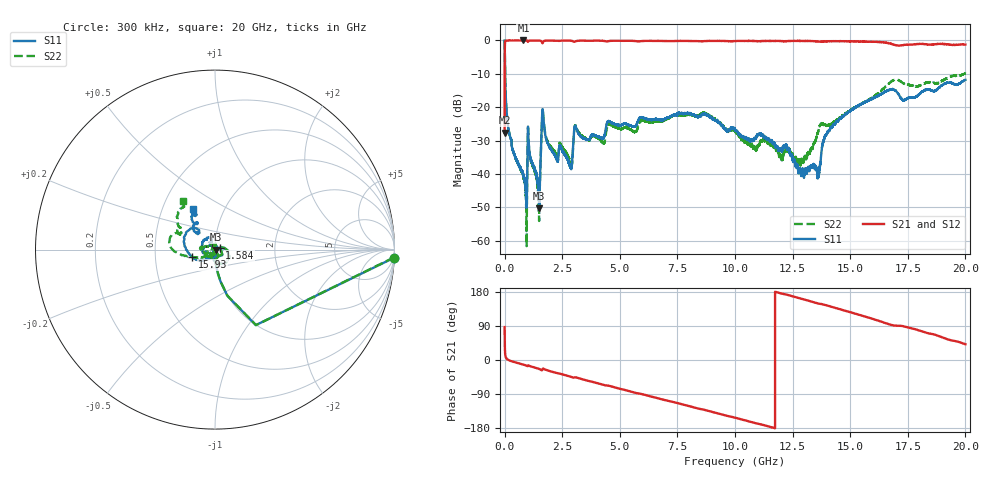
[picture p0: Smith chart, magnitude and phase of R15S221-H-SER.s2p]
!{R15S221}
!Johanson Technology Inc.
!www.johansontechnology.com
!Test Board Conditions:
!Substrate Type  RO4350B
!Substrate Thickness  20 mil
!Substrate Dk  3.66
!TL Type: GCPW
!TL Trace Width  34 mil
!TL Gap  10 mil
!Electrode orientation  Horizontal
!DUT TOPOLOGY	SERIES
!Mounting Pad LxW  26x52 mil
! Created Sat Feb  6 14:22:14 2021
# hz S ma R 50
! 2 Port Network Data from SP1.SP block
! freq  magS11  angS11  magS21  angS21  magS12  angS12  magS22  angS22
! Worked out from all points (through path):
!   20001 points, 300 kHz to 20 GHz, reference 50 ohm
!   highest |S21| = 0.00 dB at 816.3 MHz (marker M1); lowest = -27.7 dB at 300 kHz (marker M2)
!   group delay of S21, straight-line fit = 44.1 ps
!   lowest |S11| = -50.2 dB at 1.501 GHz (marker M3), VSWR 1.01, Z = 50.3 - j0.117 ohm
!   |S11| at or under -10 dB: 21.74 MHz to end of sweep
!   |S22| runs from -61.6 to 0.0 dB; largest |S21 - S12| = 0.014
!   S11 on the Smith chart (normalised r, x): 300 kHz: 2, -44; 1.584 GHz: 1.05, +0.02; 15.93 GHz: 0.77, -0.07; 20 GHz: 0.71, +0.34
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300000  0.9983 -2.6  0.0414 86.9  0.0415 87.4  0.9969 -2.5
1.073e8  0.06955 -87.6  0.9969 2.2  0.9969 2.2  0.06989 -87.4
4.003e8  0.02077 -94.3  0.9994 -5.1  0.999 -5.1  0.0206 -95.1
8.163e8  0.00948 -97.8  0.9999 -12.3  0.9984 -12.2  0.00937 -106.7
8.923e8  0.007055 -97.5  0.9982 -13.6  0.9984 -13.6  0.006714 -109.6
1.0893e9  0.02004 -101.3  0.9963 -16.1  0.9959 -16.0  0.01927 -103.2
1.5013e9  0.003086 -22.2  0.9954 -23.6  0.9954 -23.7  0.003239 -33.6
1.5843e9  0.02719 22.6  0.98 -26.2  0.9801 -26.2  0.02694 25.2
1.6943e9  0.06061 -95.3  0.9736 -23.3  0.9739 -23.3  0.06227 -89.4
2.8323e9  0.01337 -117.3  0.9924 -43.5  0.9923 -43.6  0.0153 -115.5
3.0803e9  0.0518 -110.2  0.9694 -45.6  0.9699 -45.6  0.05281 -103.1
3.3343e9  0.03567 -138.2  0.9934 -50.1  0.9929 -50.1  0.03735 -134.1
6.6673e9  0.06606 169.5  0.9849 -101.2  0.9854 -101.1  0.06213 179.5
1.00003e10  0.04616 122.4  0.9801 -152.2  0.9805 -152.2  0.04442 140.5
1.22573e10  0.02413 85.3  0.9784 172.2  0.9784 172.1  0.02541 120.2
1.27643e10  0.01065 16.6  0.9852 163.6  0.9827 163.7  0.01643 149.3
1.33343e10  0.01306 -77.4  0.9799 154.0  0.9791 153.9  0.02404 -145.3
1.36263e10  0.009404 -87.1  0.9619 148.9  0.9646 149.1  0.04513 -132.2
1.42153e10  0.04992 -114.1  0.9754 139.9  0.9749 139.8  0.05666 -146.5
1.59303e10  0.1326 -161.8  0.9549 109.4  0.9587 109.4  0.1366 -162.8
1.66673e10  0.1794 162.5  0.9114 94.5  0.9012 94.8  0.2252 -177.0
2e10  0.2564 118.9  0.8666 41.5  0.86 41.4  0.324 122.9
